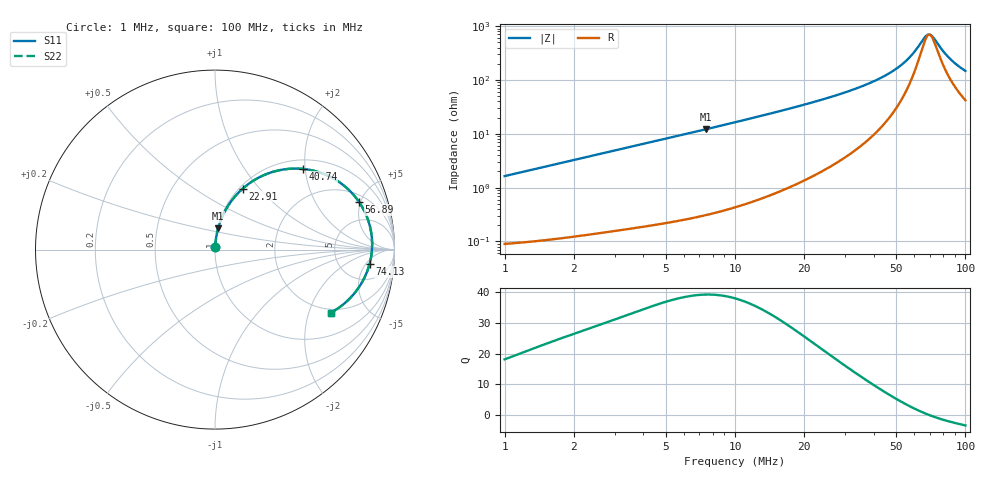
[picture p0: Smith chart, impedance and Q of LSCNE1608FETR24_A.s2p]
! LSCNE1608FETR24_A  S-PARAMETER MODEL  ( Standard Model )
! Model Generated by TAIYO YUDEN Corporation (http://www.ty-top.com)
! Version 1.0
! TAIYO YUDEN Control No. 160926
! Copyright(c) 2016 TAIYO YUDEN CO.,LTD. All Rights Reserved.
! Product Description (link to TY-COMPAS)
! https://ds.yuden.co.jp/TYCOMPAS/or/detail?pn=LSCNE1608FETR24MA&u=M
! Products Name : Inductors
! Characteristics :
!  Inductance : 0.24 [uH] , SRF(min) : - [Hz] , DC Resistance(max) : 100 [mOhm]
!  Rated Current : Saturation  2.6 [A] (dL = 30 [%]), Temp Rise  1.5 [A] (dT = 40 [degC])
!  Case Size : 1.6 x 0.8 / 0.063 x 0.031 [mm/inch] , Thickness : 0.65 / 0.026 [mm/inch]
!  (Conditions: Temperature = 25 [degC] , DC Bias Current = 0 [A])
! External Node Assignments :
!  1  o---GGG---o  2
! GND o---------o GND
! Frequency Range : 1MHz  -  100MHz  [ 402 STEP ]
# MHz S RI R 50
! Freq[MHz].  S11 Real  S11 Imag  S21 Real  S21 Imag  S12 Real  S12 Imag  S22 Real  S22 Imag
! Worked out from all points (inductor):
!   401 points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, 1 MHz to 100 MHz, reference 50 ohm
!   read as one part in series: L = 260 nH near 1.023 MHz
!   highest Q = 39.2 at 7.499 MHz (marker M1), where L = 258 nH
!   self-resonance near 69.86 MHz
!   S11 on the Smith chart (normalised r, x): 1 MHz: 1.00, +0.03; 22.91 MHz: 1.04, +0.82; 40.74 MHz: 1.21, +1.94; 56.89 MHz: 2.60, +4.84; 74.13 MHz: 10, -6; 100 MHz: 1.84, -2.82
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1  0.00117 0.0163  0.9988 -0.0163  0.9988 -0.0163  0.00117 0.0163
1.412538  0.00156 0.023  0.9984 -0.023  0.9984 -0.023  0.00156 0.023
1.905461  0.00215 0.0309  0.9978 -0.0309  0.9978 -0.0309  0.00215 0.0309
3.235937  0.00436 0.0521  0.9956 -0.0521  0.9956 -0.0521  0.00436 0.0521
5.069907  0.00884 0.0811  0.9912 -0.0811  0.9912 -0.0811  0.00884 0.0811
7.498942  0.0175 0.1191  0.9825 -0.1191  0.9825 -0.1191  0.0175 0.1191
11.88502  0.0418 0.1866  0.9582 -0.1866  0.9582 -0.1866  0.0418 0.1866
17.57924  0.0904 0.2697  0.9096 -0.2697  0.9096 -0.2697  0.0904 0.2697
22.90868  0.1544 0.3397  0.8456 -0.3397  0.8456 -0.3397  0.1544 0.3397
34.27678  0.3503 0.4405  0.6497 -0.4405  0.6497 -0.4405  0.3503 0.4405
40.73803  0.4893 0.4496  0.5107 -0.4496  0.5107 -0.4496  0.4893 0.4496
50.69907  0.7019 0.3693  0.2981 -0.3693  0.2981 -0.3693  0.7019 0.3693
56.88529  0.8023 0.2659  0.1977 -0.2659  0.1977 -0.2659  0.8023 0.2659
62.37348  0.8564 0.1545  0.1436 -0.1545  0.1436 -0.1545  0.8564 0.1545
67.6083  0.8753 0.0451  0.1247 -0.0451  0.1247 -0.0451  0.8753 0.0451
69.1831  0.8753 0.0134  0.1247 -0.0134  0.1247 -0.0134  0.8753 0.0134
70.79458  0.873 -0.0182  0.127 0.0182  0.127 0.0182  0.873 -0.0182
74.13102  0.8614 -0.0794  0.1386 0.0794  0.1386 0.0794  0.8614 -0.0794
79.43282  0.829 -0.1639  0.171 0.1639  0.171 0.1639  0.829 -0.1639
84.13951  0.7911 -0.2251  0.2089 0.2251  0.2089 0.2251  0.7911 -0.2251
92.25714  0.7171 -0.3033  0.2829 0.3033  0.2829 0.3033  0.7171 -0.3033
100  0.6451 -0.3521  0.3549 0.3521  0.3549 0.3521  0.6451 -0.3521
